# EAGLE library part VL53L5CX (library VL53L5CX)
Time-of-Flight 8x8 multizone ranging sensor with wide field of view Source: Datasheet
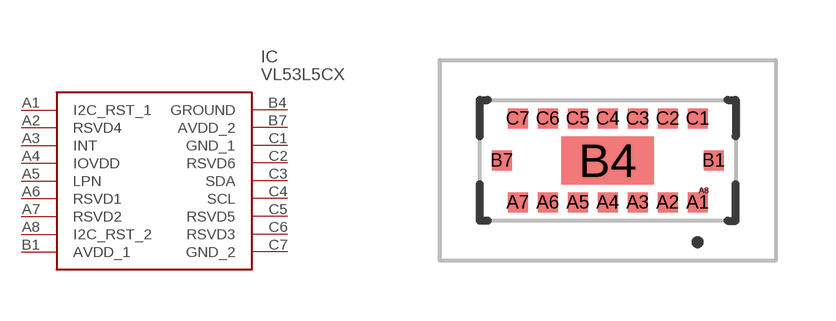
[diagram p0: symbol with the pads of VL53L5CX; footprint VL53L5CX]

Designator prefix IC

## VL53L5CX (Description: Time-of-Flight 8x8 multizone ranging sensor with wide field of view; Height: 1.55mm; Manufacturer_Name: STMicroelectronics; Manufacturer_Part_Number: VL53L5CX)  [VL53L5CX]
A1  I2C_RST_1
A2  RSVD4
A3  INT
A4  IOVDD
A5  LPN
A6  RSVD1
A7  RSVD2
A8  I2C_RST_2
B1  AVDD_1
B4  GROUND
B7  AVDD_2
C1  GND_1
C2  RSVD6
C3  SDA
C4  SCL
C5  RSVD5
C6  RSVD3
C7  GND_2

## Footprint VL53L5CX (pad centres in mm)
Optical LGA16
smd 0.5 x 0.5: A1 2.25,-1.05; A2 1.5,-1.05; A3 0.75,-1.05; A4 0,-1.05; A5 -0.75,-1.05; A6 -1.5,-1.05; A7 -2.25,-1.05; B1 2.65,0; B7 -2.65,0; C1 2.25,1.05; C2 1.5,1.05; C3 0.75,1.05; C4 0,1.05; C5 -0.75,1.05; C6 -1.5,1.05; C7 -2.25,1.05
smd 0.2 x 0.1: A8 2.4,-0.75
smd 2.316 x 1.2: B4 0,0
